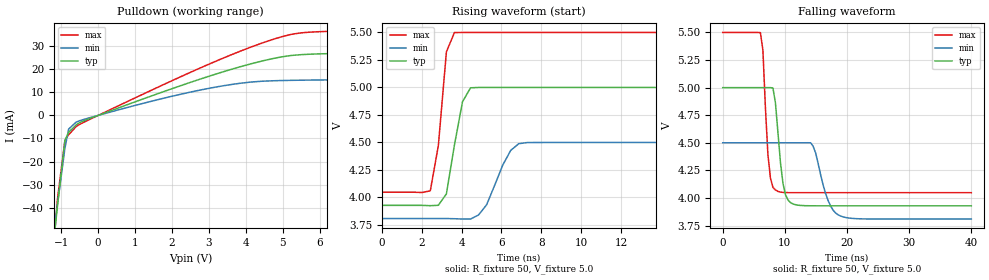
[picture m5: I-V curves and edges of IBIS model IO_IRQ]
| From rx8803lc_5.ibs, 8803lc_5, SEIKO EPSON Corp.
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[Model]   IO_IRQ
Model_type Open_drain
Enable Active-Low
Polarity Non-Inverting
C_comp   5p   4p   6p
[Temperature Range] 25   85   -40
[Voltage Range]   5.0   4.5   5.5
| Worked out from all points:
|   slope of the pulldown table from 0 to 0.75 V, typ, clamps not added: 170 ohm
|   falling waveform, R_fixture 50, V_fixture 5.0: 20-80 % time 1.08ns typ, 2.05ns min, 810ps max; typ from 5 V to 3.93 V
|   rising waveform, R_fixture 50, V_fixture 5.0: 20-80 % time 622ps typ, 983ps min, 482ps max; typ from 3.93 V to 5 V
[Pulldown]
-5V       -674.7mA   -554.2mA   -835.9mA
-1.2V     -54.21mA   -50.61mA   -55.37mA
-1.1V     -39mA      -38.39mA   -36.01mA
-900mV    -10.86mA   -14.25mA   -10.84mA
-800mV    -7.34mA    -5.937mA   -8.424mA
-500mV    -3.114mA   -2.29mA    -3.853mA
800mV     4.703mA    3.472mA    6.07mA
3.3V      18.47mA    12.59mA    24.24mA
4.2V      22.6mA     14.52mA    29.96mA
5.2V      25.88mA    15.16mA    34.98mA
5.9V      26.59mA    15.32mA    36.18mA
10V       28.2mA     16.57mA    38.06mA
[Falling Waveform]
R_fixture=50
V_fixture=5.0
V_fixture_min=4.5
V_fixture_max=5.5
0s        5V         4.5V       5.5V
6.061ns   5V         4.5V       5.499V
6.465ns   5V         4.5V       5.34V
7.273ns   5V         4.5V       4.392V
8.485ns   4.861V     4.5V       4.072V
9.697ns   4.132V     4.5V       4.05V
11.31ns   3.945V     4.5V       4.048V
14.55ns   3.929V     4.469V     4.048V
18.99ns   3.929V     3.836V     4.048V
40ns      3.928V     3.809V     4.048V
[Rising Waveform]
R_fixture=50
V_fixture=5.0
V_fixture_min=4.5
V_fixture_max=5.5
0s        3.928V     3.809V     4.048V
2.424ns   3.925V     3.809V     4.061V
2.828ns   3.929V     3.809V     4.472V
3.232ns   4.033V     3.809V     5.324V
3.636ns   4.477V     3.807V     5.499V
4.04ns    4.869V     3.804V     5.5V
4.444ns   4.997V     3.804V     5.5V
6.465ns   5V         4.428V     5.5V
7.273ns   5V         4.499V     5.5V
40ns      5V         4.5V       5.5V
[Ramp]
R_load=50
dV/dt_r   6.429E-1/5.939E-10   4.149E-1/9.366E-10   8.714E-1/3.968E-10
dV/dt_f   6.429E-1/1.057E-9   4.149E-1/2.023E-9   8.714E-1/7.472E-10
|[End   IO_IRQ
